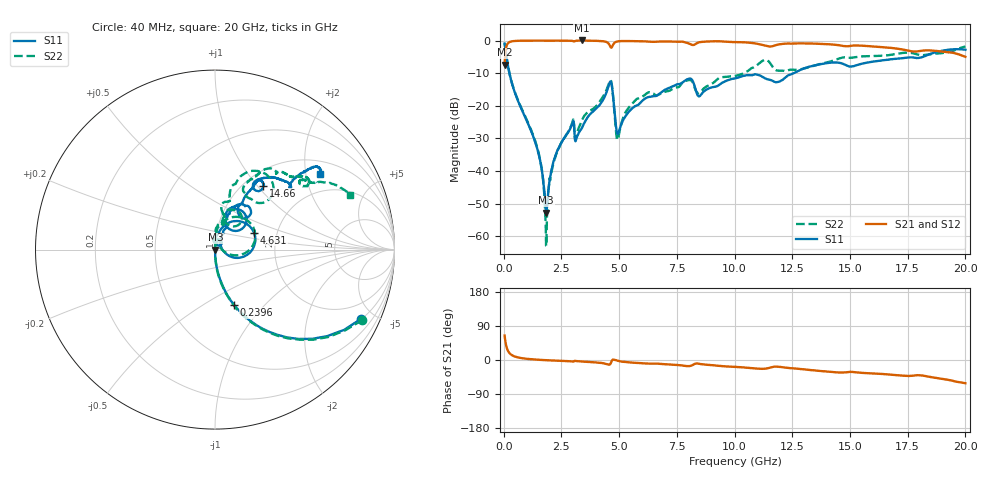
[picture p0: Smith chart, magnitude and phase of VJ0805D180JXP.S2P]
! VJ0805D180JXP
! DATE 10/29/2021  12:15
! CAPACITORS MOUNTED IN SERIES ON 25 MIL THICK MICROSTRIP SUBSTRATE
# GHz  S  MA  R  50.00
!  FREQ  S11M  S11A  S21M  S21A  S12M  S12A  S22M  S22A
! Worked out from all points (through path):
!   1601 points, 40 MHz to 20 GHz, reference 50 ohm
!   highest |S21| = 0.04 dB at 3.371 GHz (marker M1); lowest = -7.4 dB at 40 MHz (marker M2)
!   group delay of S21, straight-line fit = 8.02 ps
!   lowest |S11| = -52.8 dB at 1.836 GHz (marker M3), VSWR 1.00, Z = 50.2 - j0.0705 ohm
!   |S11| at or under -10 dB: 248.1 MHz to 12.57 GHz (12.32 GHz wide, 192 % of centre)
!   |S22| runs from -63.0 to -0.8 dB; largest |S21 - S12| = 0.0074
!   S11 on the Smith chart (normalised r, x): 40 MHz: 1.03, -4.19; 239.6 MHz: 1.00, -0.69; 4.631 GHz: 1.52, +0.31; 14.66 GHz: 1.22, +1.07; 20 GHz: 1.36, +2.42
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0.04  0.8998 -25.5  0.4289 64.5  0.4294 64.5  0.9095 -25.6
0.2396  0.3266 -70.9  0.945 19.0  0.9441 19.0  0.3301 -71.3
1.46215  0.02151 -87.3  0.9982 0.8  0.9988 0.9  0.02213 -87.7
1.6368  0.0113 -82.4  0.9987 0.2  0.9984 0.1  0.01135 -86.3
1.8364  0.002297 -17.8  0.9982 -0.5  0.9985 -0.6  0.0007144 -20.3
2.048475  0.009552 83.2  0.9977 -1.1  0.9982 -1.2  0.008746 81.5
2.3354  0.02123 84.0  0.9982 -1.9  0.9977 -1.9  0.02043 88.5
2.946675  0.05032 75.3  0.9937 -3.8  0.9947 -3.9  0.05213 87.5
3.15875  0.03208 75.0  0.9972 -2.9  0.9972 -3.0  0.03606 92.1
3.370825  0.04454 87.2  1.005 -4.0  1.005 -4.1  0.05786 100.3
4.6308  0.2371 23.6  0.7945 -9.4  0.7949 -9.5  0.247 30.3
4.95515  0.0378 27.2  0.9737 -2.5  0.9738 -2.6  0.03169 51.2
5.666225  0.09735 63.1  0.9812 -7.3  0.9817 -7.5  0.1178 87.3
6.70165  0.1485 67.7  0.968 -9.8  0.9675 -10.0  0.1475 75.2
8.04895  0.262 56.1  0.8936 -16.0  0.8934 -16.2  0.2489 59.5
8.485575  0.1406 58.5  0.9454 -10.2  0.9456 -10.4  0.1595 66.5
10.02  0.2633 65.2  0.9479 -17.9  0.9486 -18.1  0.2865 73.4
11.49205  0.2523 45.8  0.8137 -21.0  0.8134 -21.3  0.4758 46.7
13.35083  0.4069 58.6  0.9008 -26.8  0.9009 -27.0  0.4041 65.2
14.6607  0.4451 52.8  0.8336 -33.2  0.8342 -33.6  0.5486 55.6
16.68165  0.5125 52.1  0.7777 -38.2  0.7781 -38.5  0.5978 42.6
20  0.7237 35.8  0.564 -61.2  0.5637 -61.7  0.8129 22.0
